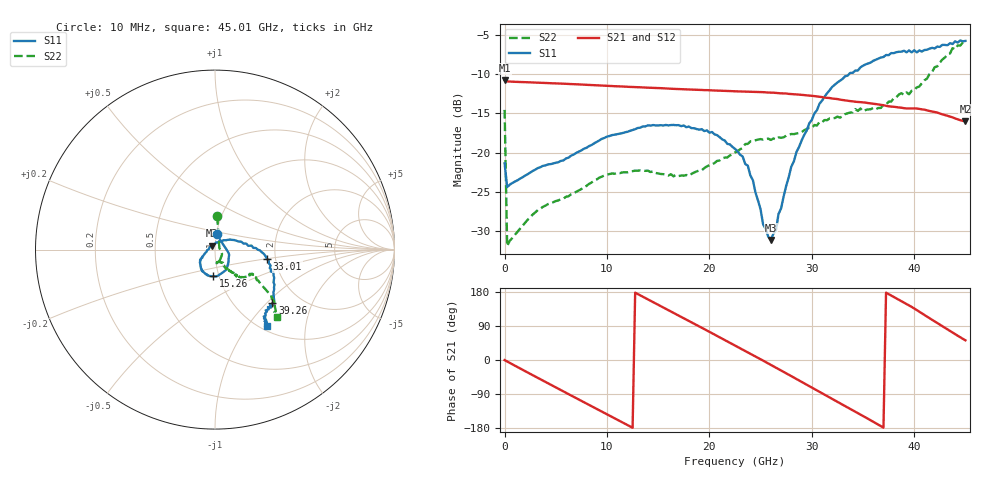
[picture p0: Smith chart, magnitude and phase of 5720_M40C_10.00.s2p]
! Device:  ADRF5720
! Description: 0.5dB LSB GaAs MMIC 6-bit Digital Attenuator
! Frequency:  0.000009 -  40 GHz
! Ports:
!	RF1	= Port 1
!	RF2	= Port 2
! Vdd:  3.3 Volt
! Vss:  -3.3 Volt
! Control:  0/3.3 Volt
! State:  10.00 dB attenuation
! Data:  The device was measured using G-S-G Probes on a matrix board.
!  Data was collected using an calibrated 4 port network analyzer.
!  The reference plane for this measurement is at the launchers.
! Note:  Analog Devices supplies this data as a sample of measured data
!  for this product.  Your particular data for this product may vary.
!  Data was taken at -40 degrees C.
!  Analog Devices reserves the right to change this data at anytime.
# GHZ S DB R 45.0
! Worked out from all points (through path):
!   181 points, 10 MHz to 45.01 GHz, reference 45 ohm
!   highest |S21| = -10.77 dB at 10 MHz (marker M1); lowest = -16.0 dB at 45.01 GHz (marker M2)
!   group delay of S21, straight-line fit = 40.8 ps
!   lowest |S11| = -31.1 dB at 26.01 GHz (marker M3), VSWR 1.06, Z = 43.4 + j1.88 ohm
!   |S11| at or under -10 dB: start of sweep to 33.65 GHz
!   |S22| runs from -31.9 to -5.9 dB; largest |S21 - S12| = 0.0011
!   S11 on the Smith chart (normalised r, x): 10 MHz: 1.00, +0.17; 15.26 GHz: 0.94, -0.29; 33.01 GHz: 1.80, -0.21; 39.26 GHz: 1.47, -1.07; 45.01 GHz: 1.06, -1.24
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0.01  -21.37 84.2  -10.77 -0.2  -10.79 -0.2  -14.56 86.3
0.26  -24.40 6.9  -10.93 -4.0  -10.95 -4.0  -31.93 16.5
4.26  -21.50 -20.4  -11.15 -61.6  -11.17 -61.6  -26.56 -33.9
7.76  -19.51 -45.8  -11.34 -111.5  -11.36 -111.5  -24.41 -60.2
11.51  -17.52 -69.3  -11.58 -164.6  -11.60 -164.7  -22.53 -76.6
15.26  -16.51 -93.9  -11.79 142.1  -11.81 142.0  -22.73 -82.1
19.01  -17.08 -117.4  -12.01 88.7  -12.03 88.6  -22.28 -66.4
22.76  -19.82 -144.7  -12.20 34.8  -12.22 34.7  -19.84 -60.6
23.76  -21.67 -150.5  -12.25 20.3  -12.27 20.2  -18.90 -60.9
25.26  -29.18 176.1  -12.30 -1.7  -12.33 -1.8  -18.36 -59.5
26.01  -31.14 128.7  -12.36 -12.8  -12.39 -12.9  -18.39 -59.0
26.51  -29.89 90.0  -12.40 -20.3  -12.43 -20.5  -18.32 -59.6
26.76  -27.83 80.5  -12.43 -24.0  -12.46 -24.1  -18.07 -57.5
28.01  -21.78 39.8  -12.54 -42.6  -12.56 -42.7  -17.63 -58.0
30.26  -15.02 10.9  -12.80 -76.6  -12.83 -76.7  -16.49 -54.9
33.01  -10.62 -10.2  -13.30 -117.9  -13.33 -118.0  -15.36 -50.5
35.51  -8.64 -27.7  -13.69 -155.3  -13.71 -155.5  -14.50 -49.2
37.76  -7.32 -40.0  -14.14 170.4  -14.16 170.2  -13.50 -46.3
39.26  -7.22 -42.7  -14.38 147.9  -14.40 147.7  -12.33 -36.2
40.51  -6.98 -48.0  -14.44 127.4  -14.46 127.1  -11.58 -35.0
42.01  -6.73 -54.0  -14.83 101.7  -14.85 101.5  -9.12 -37.9
45.01  -5.77 -56.1  -16.02 51.9  -16.06 51.8  -5.90 -47.4
